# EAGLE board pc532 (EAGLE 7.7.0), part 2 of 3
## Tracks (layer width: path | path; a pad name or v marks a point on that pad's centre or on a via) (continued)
!SD0 (continued)
  Bottom 0.305: RES18.1 300.99,114.3 300.99,125.09 302.26,126.36 CONN16.2 300.99,130.81 300.99,133.35 288.93,145.41 286.38,145.41 CONN15.A14 284.48,149.86 283.21,151.13 283.21,163.83 284.48,165.1 CONN14.A14 284.48,170.18 283.21,171.45 283.21,184.15 284.48,185.42 CONN13.A14 284.48,190.5 283.21,191.77 283.21,204.47 284.48,205.74 CONN12.A14
!SD1
  Top 0.305: RES18.2 289.56,105.41 289.56,95.25 288.29,93.98 U57.9
  Bottom 0.305: RES18.2 299.72,115.57 CONN16.4 298.45,130.81 298.45,133.35 287.65,144.15 285.12,144.15 CONN15.A15 281.94,149.86 280.67,151.13 280.67,163.83 281.94,165.1 CONN14.A15 281.94,170.18 280.67,171.45 280.67,184.15 281.94,185.42 CONN13.A15 281.94,190.5 280.67,191.77 280.67,204.47 281.94,205.74 CONN12.A15
!SD2
  Route2 0.305: RES18.3 292.1,107.95 292.1,90.17 U57.8
  Bottom 0.305: RES18.3 297.18,115.57 CONN16.6 295.91,130.81 295.91,133.35 286.38,142.88 283.85,142.88 CONN15.A16 279.4,149.86 278.13,151.13 278.13,163.83 279.4,165.1 CONN14.A16 279.4,170.18 278.13,171.45 278.13,184.15 279.4,185.42 CONN13.A16 279.4,190.5 278.13,191.77 278.13,204.47 279.4,205.74 CONN12.A16
!SD3
  Route2 0.305: RES18.4 289.56,107.95 289.56,92.71 U57.7
  Bottom 0.305: RES18.4 294.64,115.57 CONN16.8 293.37,130.81 293.37,133.35 285.12,141.6 282.57,141.6 CONN15.A17 276.86,149.86 275.59,151.13 275.59,163.83 276.86,165.1 CONN14.A17 276.86,170.18 275.59,171.45 275.59,184.15 276.86,185.42 CONN13.A17 276.86,190.5 275.59,191.77 275.59,204.47 276.86,205.74 CONN12.A17
!SD4
  Route2 0.305: U57.6 294.64,90.17 294.64,110.49 293.37,111.76 288.29,111.76 RES18.5
  Bottom 0.305: RES18.5 292.1,115.57 CONN16.10 290.83,130.81 290.83,133.35 283.85,140.34 281.31,140.34 CONN15.A18 274.32,149.86 273.05,151.13 273.05,163.83 274.32,165.1 CONN14.A18 274.32,170.18 273.05,171.45 273.05,184.15 274.32,185.42 CONN13.A18 274.32,190.5 273.05,191.77 273.05,204.47 274.32,205.74 CONN12.A18
!SD5
  Top 0.305: RES18.6 287.02,105.41 287.02,88.27 288.93,86.36 U57.5
  Bottom 0.305: RES18.6 289.56,115.57 CONN16.12 288.29,130.81 288.29,133.35 282.57,139.06 280.04,139.06 CONN15.A19 271.78,149.86 270.51,151.13 270.51,163.83 271.78,165.1 CONN14.A19 271.78,170.18 270.51,171.45 270.51,184.15 271.78,185.42 CONN13.A19 271.78,190.5 270.51,191.77 270.51,204.47 271.78,205.74 CONN12.A19
!SD6
  Bottom 0.305: U57.4 294.64,87.63 294.64,100.33 RES18.13 287.02,107.95 282.57,107.95 281.94,108.58 281.94,109.86 287.02,114.94 CONN16.14 285.75,130.81 285.75,133.35 281.31,137.79 278.76,137.79 CONN15.A20 269.24,149.86 267.97,151.13 267.97,163.83 269.24,165.1 CONN14.A20 269.24,170.18 267.97,171.45 267.97,184.15 269.24,185.42 CONN13.A20 269.24,190.5 267.97,191.77 267.97,204.47 269.24,205.74 CONN12.A20
!SD7
  Bottom 0.305: U57.3 292.1,85.09 292.1,100.33 RES18.12 285.75,106.68 280.67,106.68 278.76,108.58 278.76,110.49 284.48,116.2 CONN16.16 283.21,130.81 283.21,133.35 280.04,136.53 277.5,136.53 CONN15.A21 266.7,149.86 265.43,151.13 265.43,163.83 266.7,165.1 CONN14.A21 266.7,170.18 265.43,171.45 265.43,184.15 266.7,185.42 CONN13.A21 266.7,190.5 265.43,191.77 265.43,204.47 266.7,205.74 CONN12.A21
!SD10
  Route2 0.305: CONN1.4 160.02,8.89 160.02,26.67 U41.39
  Bottom 0.305: U41.39 151.13,27.94 RES14.4
!SD20
  Top 0.305: U41.40 160.02,26.67 157.48,26.67 RES14.1
  Route2 0.305: CONN1.6 154.94,8.89 154.94,21.59 RES14.1
!SD30
  Route2 0.305: CONN1.8 152.4,8.89 152.4,21.59 RES14.2
  Bottom 0.305: U41.41 153.67,25.4 RES14.2
!SD40
  Route2 0.305: CONN1.10 149.86,8.89 149.86,21.59 RES14.3
  Bottom 0.305: U41.42 160.02,26.67 152.4,26.67 RES14.3
!SD50
  Bottom 0.305: CONN1.12 149.86,8.89 149.86,13.34 151.13,14.61 RES14.13 154.31,18.41 156.84,18.41 158.75,20.32 U41.44
!SD60
  Bottom 0.305: CONN1.14 147.32,8.89 147.32,13.34 148.59,14.61 RES14.12 153.03,19.68 155.57,19.68 157.48,21.59 160.02,21.59 U41.45
!SD70
  Top 0.305: U41.46 162.56,19.05 149.86,19.05 RES14.11
  Bottom 0.305: CONN1.16 144.78,8.89 144.78,13.34 146.05,14.61 RES14.11
!SDONE
  Top 0.305: U35.C6 157.48,163.83 157.48,170.81 156.84,171.45 R4.1 140.97,176.53 U24.J11
!SDP
  Bottom 0.305: CONN12.A22 264.16,205.74 262.89,204.47 262.89,191.77 264.16,190.5 CONN13.A22 264.16,185.42 262.89,184.15 262.89,171.45 264.16,170.18 CONN14.A22 264.16,165.1 262.89,163.83 262.89,151.13 264.16,149.86 CONN15.A22 276.23,135.25 278.76,135.25 280.67,133.35 280.67,130.81 CONN16.18 281.94,115.57 277.5,111.12 277.5,107.95 280.04,105.41 284.48,105.41 RES18.11 288.29,96.52 285.75,93.98 U57.11
!SDP0
  Bottom 0.305: CONN1.18 142.24,8.89 142.24,13.34 143.51,14.61 RES14.10 149.22,20.95 154.94,20.95 158.12,24.13 162.56,24.13 U41.47
!SIO
  Top 0.305: RES17.6 256.54,104.14 261.62,104.14 262.89,102.87 262.89,99.06 271.78,90.17 276.86,90.17 U57.19
  Bottom 0.305: RES17.6 241.3,119.38 CONN16.50 240.03,130.81 240.03,142.24 241.3,143.51 CONN15.A31 241.3,149.86 240.03,151.13 240.03,163.83 241.3,165.1 CONN14.A31 241.3,170.18 240.03,171.45 240.03,184.15 241.3,185.42 CONN13.A31 241.3,190.5 240.03,191.77 240.03,204.47 241.3,205.74 CONN12.A31
!SIO0
  Top 0.305: U41.33 123.19,35.56 RES12.6
  Bottom 0.305: CONN1.50 101.6,8.89 101.6,13.97 RES12.6
!SLOW
  Route15 0.305: U38.6 165.1,114.3 167.64,114.3 U37.19
!SLOWC
  Route15 0.305: U50.2 249.56,99.69 300.36,99.69 304.17,103.5 306.7,103.5 U58.4
!SLOWS  (via drill 0.33)
  Top 0.305: v188.59,104.78 184.78,108.58 166.37,108.58 165.1,109.86 165.1,111.76 160.66,116.2 158.12,116.2 U37.13
  Route15 0.305: U58.5 307.98,107.31 304.17,107.31 301.62,104.78 v188.59,104.78
!SMSG
  Bottom 0.305: U57.21 276.86,87.63 274.95,87.63 273.05,89.53 273.05,97.79 RES17.2 251.46,119.38 CONN16.42 250.19,130.81 250.19,142.24 251.46,143.51 CONN15.A27 251.46,149.86 250.19,151.13 250.19,163.83 251.46,165.1 CONN14.A27 251.46,170.18 250.19,171.45 250.19,184.15 251.46,185.42 CONN13.A27 251.46,190.5 250.19,191.77 250.19,204.47 251.46,205.74 CONN12.A27
!SMSG0
  Bottom 0.305: CONN1.42 111.76,8.89 111.76,12.06 114.3,14.61 114.3,16.51 RES12.2 129.54,31.75 154.94,31.75 157.48,34.29 160.02,34.29 U41.34
!SPC
  Bottom 0.305: U35.R9 185.42,171.45 177.8,171.45 175.26,173.99 148.59,173.99 147.32,175.26 135.89,175.26 U24.J10
!SREQ
  Bottom 0.305: U57.22 260.35,99.06 260.35,102.87 RES17.5 243.84,119.38 CONN16.48 242.57,130.81 242.57,142.24 243.84,143.51 CONN15.A30 243.84,149.86 242.57,151.13 242.57,163.83 243.84,165.1 CONN14.A30 243.84,170.18 242.57,171.45 242.57,184.15 243.84,185.42 CONN13.A30 243.84,190.5 242.57,191.77 242.57,204.47 243.84,205.74 CONN12.A30
!SREQ0
  Route15 0.305: RES12.5 113.03,35.56 120.65,43.18 U41.27
  Bottom 0.305: CONN1.48 104.14,8.89 104.14,13.97 RES12.5
!SRST
  Bottom 0.305: U57.18 275.59,97.79 RES17.1 254,119.38 CONN16.40 252.73,130.81 252.73,142.24 254,143.51 CONN15.A26 254,149.86 252.73,151.13 252.73,163.83 254,165.1 CONN14.A26 254,170.18 252.73,171.45 252.73,184.15 254,185.42 CONN13.A26 254,190.5 252.73,191.77 252.73,204.47 254,205.74 CONN12.A26
!SRST0
  Top 0.305: RES12.11 120.65,20.32 123.83,20.32 137.79,34.29 160.02,34.29 U41.36
  Bottom 0.305: CONN1.40 114.3,8.89 114.3,12.06 115.57,13.34 RES12.11
!SSEL
  Top 0.305: U57.14 281.94,90.17 281.94,92.08 280.04,93.98 274.32,93.98 RES17.3
  Bottom 0.305: RES17.3 248.92,119.38 CONN16.44 247.65,130.81 247.65,142.24 248.92,143.51 CONN15.A28 248.92,149.86 247.65,151.13 247.65,163.83 248.92,165.1 CONN14.A28 248.92,170.18 247.65,171.45 247.65,184.15 248.92,185.42 CONN13.A28 248.92,190.5 247.65,191.77 247.65,204.47 248.92,205.74 CONN12.A28
!SSEL0
  Route15 0.305: RES12.3 118.11,38.1 120.65,40.64 U41.29
  Bottom 0.305: CONN1.44 109.22,8.89 109.22,12.06 111.76,14.61 111.76,16.51 RES12.3
!TXD0
  Top 0.305: U47.14 U48.33
!TXD1
  Route2 0.305: U48.13 201.93,26.67 201.93,16.51 U49.14
!TXD2
  Top 0.305: U51.14 U52.33
!TXD3
  Route2 0.305: U52.13 236.22,26.67 236.22,16.51 U53.14
!TXD4
  Top 0.305: U54.14 U55.33
!TXD5
  Route2 0.305: U55.13 270.51,26.67 270.51,16.51 U56.14
!TXD6
  Top 0.305: U59.14 U60.33
!TXD7
  Route2 0.305: U60.13 304.8,26.67 304.8,16.51 U61.14
!WEA
  Route2 0.305: U18.6 58.42,73.66 RES7.5
!WEAB
  Route2 0.305: U18.9 63.5,66.04 U18.5
  Bottom 0.305: U18.5 65.41,69.22 107.95,69.22 117.47,78.74 117.47,88.27 120.02,90.81 126.36,90.81 U30.11
!WEAR
  Route2 0.305: U6.21 50.8,139.7 50.8,127 U8.21 50.8,124.46 50.8,111.76 U10.21 50.8,109.22 50.8,96.52 U12.21 50.8,93.98 50.8,85.09 RES7.6
!WEB
  Route2 0.305: RES7.7 53.34,68.58 U18.8
!WEBR
  Route2 0.305: RES7.8 49.53,81.28 U13.21 49.53,92.71 48.26,93.98 48.26,96.52 49.53,97.79 U11.21 49.53,107.95 48.26,109.22 48.26,111.76 49.53,113.03 U9.21 49.53,123.19 48.26,124.46 48.26,127 49.53,128.27 U7.21
!WR
  Top 0.305: U46.31 231.14,63.5 252.09,63.5 255.27,60.33 255.27,31.75 252.73,29.21 233.68,29.21 U52.9 | U38.18 172.72,99.06 172.72,57.15 170.18,54.61 170.18,44.45 U41.21
  Route2 0.305: U41.21 168.91,39.37 179.07,29.21 196.85,29.21 U48.9
  Route15 0.305: U48.9 199.39,26.67 231.14,26.67 U52.9 233.68,26.67 265.43,26.67 U55.9 267.97,26.67 299.72,26.67 U60.9 | U46.31 232.41,74.93 279.4,74.93 U57.32
+5V
  pour Power (rank 6): 0,215.9 0,58.42 12.7,58.42 12.7,0 342.9,0 342.9,215.9
+12V
  Top 0.813: CONN12.B9 297.18,210.82 323.21,210.82 327.02,207.01 327.02,198.12 | 327.02,198.12 300.99,198.12 297.18,194.31 CONN13.B9 | 327.02,198.12 327.02,180.34 | 327.02,180.34 C68.+ | 327.02,180.34 327.02,177.8 | 327.02,177.8 300.99,177.8 297.18,173.99 CONN14.B9 | 327.02,177.8 327.02,157.48 | 327.02,157.48 300.99,157.48 297.18,153.67 CONN15.B9 | 327.02,157.48 327.02,92.08 322.58,87.63 322.58,71.75 325.75,68.58 325.75,45.72 323.85,43.81 323.85,31.11 325.12,29.84 325.12,14.61 322.58,12.06 313.06,12.06 310.31,9.32 CONN11.P8-3
  Route15 0.305: 275.59,59.69 U54.1
  Route15 0.406: U56.1 278.13,24.13 309.88,24.13 U61.1 311.15,20.32 309.88,19.05 309.88,12.7 310.31,12.27 CONN11.P8-3 | U49.1 209.55,24.13 241.3,24.13 U53.1 248.92,16.51 248.92,13.97 252.73,10.16 C59.+ | U47.1 209.55,59.69 241.3,59.69 U51.1 243.84,59.69 275.59,59.69 | U54.1 278.13,59.69 309.88,59.69 U59.1
  Route15 0.813: C59.+ 260.99,10.16 262.89,8.26 265.43,8.26 270.51,3.17 308.61,3.17 310.31,4.88 CONN11.P8-3
  Bottom 0.406: U61.1 316.23,27.94 316.23,53.34 U59.1
+V  (via drill 0.33)
  Top 0.305: U35.D11 U35.C11 | U35.C11 U35.B11 | U35.B11 U35.A11 | U35.C12 U35.C11 | U35.C11 U35.C10 | U35.B12 U35.B11 | U35.B11 U35.B10 | U32.4 125.73,68.58 U32.10 | U31.4 129.54,82.55 134.62,82.55 U31.1 | v226.06,111.76 226.06,103.5 228.6,100.97 v228.6,92.71
  Route2 0.305: U35.N12 177.16,177.8 174.62,175.26 U35.D11 | U35.S14 205.74,182.88 224.79,163.83 224.79,144.78 | 224.79,144.78 224.79,142.24 U43.22 | 224.79,144.78 227.33,142.24 227.33,113.03 v226.06,111.76 | U30.10 127,87.63 127,85.09 U31.4 127,82.55 127,72.39 U32.4 | U46.28 220.34,70.48 220.34,74.93 224.79,79.38 224.79,84.45 228.6,88.27 v228.6,92.71 | RES13.2 179.07,86.36 v179.07,106.68 179.07,132.08 175.26,135.89 173.99,135.89 U36.2
  Route15 0.305: U30.5 127,95.25 127,90.17 U30.10 | U35.R14 185.42,181.61 183.51,181.61 182.88,180.97 182.88,179.07 | 182.88,179.07 U35.N12 | U35.B12 U35.B13 | U35.D11 160.02,173.99 160.02,163.83 U35.D6 | RES13.2 162.56,72.39 160.02,72.39 RES13.4 RES13.5 154.94,72.39 129.54,72.39 U32.4 | v179.07,106.68 203.84,106.68 205.74,108.58 222.88,108.58 v226.06,111.76 | U50.1 245.11,92.71 v228.6,92.71 | U24.B7 125.73,195.58 125.73,201.93 128.27,204.47 137.16,204.47 149.86,191.77 149.86,184.15 U35.A14 | 182.88,179.07 U35.P12
  Bottom 0.305: U26.1 135.89,151.13 135.89,156.21 140.97,161.29 157.48,161.29 U35.D6 | U33.6 U32.10 | U35.R14 U35.S14 | U35.B13 U35.A13 U35.A14 | U24.A5 123.19,195.58 | 123.19,195.58 125.73,195.58 U24.B7 | U24.B5 123.19,195.58
-12V
  Top 0.406: U61.8 292.1,24.13 292.1,57.15 U59.8
  Route2 0.61: 304.17,3.17 306.35,5.36 CONN11.P8-4
  Route2 0.635: C60.- 268.61,5.08 270.51,3.17 304.17,3.17
  Route15 0.406: U56.8 260.35,21.59 290.83,21.59 | 290.83,21.59 292.1,21.59 U61.8 | U47.8 191.77,57.15 223.52,57.15 U51.8 226.06,57.15 257.81,57.15 U54.8 260.35,57.15 292.1,57.15 U59.8 | 290.83,21.59 290.83,15.24 293.37,12.7 302.26,12.7 306.35,8.61 CONN11.P8-4
  Bottom 0.406: U56.8 257.81,21.59 226.06,21.59 U53.8 223.52,21.59 191.77,21.59 U49.8
  Bottom 0.813: CONN12.B7 302.26,210.82 323.21,210.82 327.02,207.01 327.02,198.12 | 327.02,198.12 305.44,198.12 302.26,194.94 CONN13.B7 | 327.02,198.12 327.02,194.31 | 327.02,194.31 C67.- | 327.02,194.31 327.02,177.8 | 327.02,177.8 306.07,177.8 302.26,173.99 CONN14.B7 | 327.02,177.8 327.02,157.48 | 327.02,157.48 306.07,157.48 302.26,153.67 CONN15.B7 | 327.02,157.48 327.02,92.08 322.58,87.63 322.58,71.12 331.47,62.23 331.47,15.88 327.66,12.06 309.25,12.06 306.35,9.17 CONN11.P8-4
_STERM
  Top 0.813: D3.A F2.1
_STERM0
  Top 0.813: D1.A F1.1
A0  (via drill 0.33)
  Route2 0.305: U44.10 204.47,132.08 204.47,98.42 v203.84,97.79
  Route15 0.305: U35.R6 187.96,161.29 190.5,161.29 201.93,149.86 201.93,139.7 205.74,135.89 U44.10
  Bottom 0.305: v203.84,97.79 214.63,97.79 U45.3
A1
  Route2 0.305: U45.5 210.82,97.79 207.01,101.6 207.01,132.08 U44.9
  Route15 0.305: U35.S5 191.77,157.48 191.77,147.32 204.47,134.62 204.47,132.72 205.1,132.08 207.01,132.08 U44.9
A2
  Route2 0.305: U27.2 142.88,141.6 142.88,151.76 149.86,158.75 165.1,158.75 167.64,161.29 182.88,161.29 U35.P6 | U44.8 210.82,129.54 212.09,128.27 212.09,92.71 U45.9
  Route15 0.305: U44.8 204.47,139.7 204.47,149.86 190.5,163.83 185.42,163.83 U35.P6
A3
  Top 0.305: U27.5 133.35,139.7 138.43,139.7 146.69,147.96 164.47,147.96 165.1,148.59 165.1,156.21 167.64,158.75 187.96,158.75 U35.S4
  Route2 0.305: U45.11 217.17,92.71 217.17,101.6 214.63,104.14 214.63,129.54 213.36,130.81 U44.7
  Route15 0.305: U35.S4 190.5,156.21 190.5,147.32 201.93,135.89 201.93,132.08 203.2,130.81 210.82,130.81 U44.7
A4  (via drill 0.33)
  Top 0.305: U27.11 125.73,129.54 128.27,132.08 138.43,132.08 140.34,133.99 140.34,135.25 141.6,136.53 143.51,136.53 144.15,137.16 144.15,143.51 147.32,146.69 v159.38,146.69
  Route2 0.305: U45.13 219.71,90.17 219.71,129.54 U44.6
  Route15 0.305: v159.38,146.69 163.19,146.69 165.1,148.59 165.1,156.21 167.64,158.75 185.42,158.75 U35.R5 187.96,158.75 187.96,148.59 199.39,137.16 199.39,132.08 201.93,129.54 212.09,129.54 U44.6
A5  (via drill 0.33)
  Top 0.305: v187.96,142.24 187.96,137.16 181.61,130.81 181.61,127 177.8,123.19 163.83,123.19 162.56,121.92 146.05,121.92 144.15,123.83 136.53,123.83 U27.14
  Route2 0.305: U44.5 222.25,129.54 222.25,114.3 220.98,113.03 U45.1
  Bottom 0.305: U35.S3 187.96,153.67 v187.96,142.24 190.5,139.7 212.09,139.7 U44.5
A6  (via drill 0.33)
  Top 0.305: v155.57,142.88 153.67,140.97 v145.41,140.97
  Route2 0.305: U33.3 132.08,57.15 130.18,57.15 129.54,57.78 129.54,59.69 132.08,62.23 132.08,64.77 134.62,67.31 134.62,73.03 132.08,75.56 132.08,85.09 129.54,87.63 129.54,97.79 132.08,100.33 132.08,104.14 134.62,106.68 134.62,115.57 135.89,116.84 U28.2
  Route15 0.305: U28.2 140.34,126.36 140.34,128.91 144.15,132.72 144.15,139.7 v145.41,140.97 | v155.57,142.88 155.57,146.05 157.48,147.96 161.93,147.96 162.56,148.59 162.56,156.21 167.64,161.29 182.88,161.29 U35.P5
  Bottom 0.305: U44.4 214.63,139.7 214.63,142.24 213.36,143.51 193.04,143.51 191.77,144.78 191.77,157.48 190.5,158.75 185.42,158.75 U35.P5
A7  (via drill 0.33)
  Top 0.305: v156.84,144.78 v147.32,144.78
  Route15 0.305: v156.84,144.78 163.83,144.78 167.64,148.59 167.64,155.57 168.28,156.21 185.42,156.21 U35.R4 | v147.32,144.78 146.05,144.78 140.34,139.06 140.34,133.99 138.43,132.08 133.35,132.08 129.54,128.27 129.54,123.19 U28.5
  Bottom 0.305: U35.R4 185.42,156.21 185.42,148.59 186.69,147.32 186.69,140.97 189.23,138.43 212.09,138.43 214.63,135.89 214.63,132.08 215.9,130.81 220.98,130.81 U44.3
A8  (via drill 0.33)
  Top 0.305: U44.25 222.25,116.84 224.16,116.84 224.79,117.47 224.79,119.38 222.25,121.92 222.25,142.24 219.71,144.78 196.85,144.78 U35.S2 | v182.25,138.43 v189.23,145.41
  Route15 0.305: v182.25,138.43 175.9,132.08 175.9,130.18 174.62,128.91 161.93,128.91 U37.7
  Bottom 0.305: U35.S2 190.5,151.13 190.5,146.69 v189.23,145.41 | U28.11 127,113.03 129.54,113.03 132.08,110.49 132.08,107.95 133.35,106.68 139.06,106.68 140.34,107.95 140.34,110.49 141.6,111.76 152.4,111.76 157.48,116.84 157.48,124.46 U37.7
A9  (via drill 0.33)
  Top 0.305: U28.14 135.89,116.84 144.78,116.84 148.59,120.65 179.07,120.65 v181.61,123.19 | U35.R3 187.96,153.67 190.5,153.67 198.12,146.05 220.98,146.05 224.79,142.24 224.79,121.92 227.33,119.38 227.33,117.47 225.43,115.57 220.98,115.57 U44.24
  Bottom 0.305: v181.61,123.19 186.69,123.19 195.58,114.3 214.63,114.3 U44.24
A10  (via drill 0.33)
  Top 0.305: v182.88,129.54 182.88,121.92 180.34,119.38 149.86,119.38 142.24,111.76 138.43,111.76 U29.2
  Bottom 0.305: U44.21 204.47,124.46 190.5,124.46 185.42,129.54 184.15,129.54 | 184.15,129.54 v182.88,129.54 | 184.15,129.54 184.15,147.32 182.88,148.59 182.88,156.21 U35.P4
A11  (via drill 0.33)
  Top 0.305: U29.5 130.18,107.31 142.88,107.31 144.15,106.05 148.59,106.05 149.86,107.31 v173.99,107.31
  Bottom 0.305: U44.23 213.36,115.57 208.28,115.57 207.01,116.84 207.01,119.38 204.47,121.92 190.5,121.92 186.69,125.73 180.34,125.73 | 180.34,125.73 180.34,110.49 177.16,107.31 v173.99,107.31 | U35.N4 180.34,156.21 180.34,125.73
A12  (via drill 0.33)
  Top 0.305: U35.R2 185.42,153.67 185.42,155.57 186.06,156.21 190.5,156.21 199.39,147.32 222.25,147.32 227.33,142.24 227.33,134.62 U44.2
  Route2 0.305: U29.11 132.08,107.95 132.08,115.57 134.62,118.11 134.62,123.19 135.89,124.46 143.51,124.46 146.69,127.64 | 146.69,127.64 J1.3 | 146.69,127.64 147.32,128.27 153.67,128.27 154.94,129.54 154.94,131.44 155.57,132.08 165.1,132.08 v166.37,133.35
  Route15 0.305: U35.R2 185.42,151.13 185.42,149.22 179.71,143.51 171.45,143.51 167.64,139.7 167.64,135.89 166.37,134.62 v166.37,133.35
A13
  Top 0.305: U36.3 168.91,140.97 175.26,147.32 186.69,147.32 U35.S1 195.58,143.51 218.44,143.51 219.71,142.24 219.71,121.92 U44.26
  Route2 0.305: U36.3 165.1,134.62 157.48,134.62 156.21,133.35 153.67,133.35 152.4,132.08 152.4,130.18 151.76,129.54 150.5,129.54 147.96,132.08 128.27,132.08 U27.6
A14  (via drill 0.33)
  Top 0.305: U36.4 169.54,135.25 v182.25,135.25 | U27.10 123.19,129.54 127,133.35 131.44,133.35 132.08,133.99 132.08,135.89 134.62,138.43 v142.88,138.43
  Route2 0.305: U35.N3 180.34,156.21 149.86,156.21 144.15,150.5 144.15,139.7 v142.88,138.43
  Route15 0.305: U35.N3 180.34,153.67 180.34,149.22 175.9,144.78 171.45,144.78 166.37,139.7 U36.4 | v182.25,135.25 187.96,135.25 200.03,123.19 220.98,123.19 U44.27
A15  (via drill 0.33)
  Top 0.305: U27.13 132.08,128.27 153.67,128.27 154.94,129.54 v154.94,134.62 | U36.5 173.99,148.59 185.42,148.59 U35.R1
  Route2 0.305: v154.94,134.62 156.21,135.89 161.29,135.89 U36.5
A16
  Route2 0.305: U35.P1 184.15,148.59 176.53,140.97 163.83,140.97 U36.6
  Bottom 0.305: U28.3 134.62,123.19 134.62,135.89 138.43,139.7 160.02,139.7 U36.6
A17
  Route15 0.305: U35.M3 177.8,153.67 177.8,151.76 177.16,151.13 175.9,151.13 175.26,150.5 175.26,149.22 173.35,147.32 171.45,147.32 165.1,140.97 161.29,140.97 U36.7
  Bottom 0.305: U28.6 128.27,119.38 138.43,119.38 140.34,121.28 140.34,129.54 145.41,134.62 152.4,134.62 153.67,135.89 156.21,135.89 U36.7
A18  (3 unrouted)
  Top 0.305: U36.8 154.94,139.7 150.5,139.7 149.86,139.06 149.86,135.89 148.59,134.62 144.78,134.62 140.97,130.81 129.54,130.81 127,128.27 127,118.11 U28.10
  Route2 0.305: U36.8 163.19,145.41 176.53,145.41 180.97,149.86 U35.N2
A19
  Top 0.305: U28.13 130.81,116.84 129.54,118.11 129.54,128.27 130.81,129.54 147.32,129.54 153.67,135.89 U36.9
  Route2 0.305: U36.9 154.94,137.16 160.02,137.16 160.02,139.7 164.47,144.15 177.8,144.15 182.88,149.22 182.88,151.13 U35.N1
A20
  Route2 0.305: U35.M1 175.9,146.69 163.19,146.69 157.48,140.97 153.67,140.97 152.4,139.7 152.4,134.62 151.13,133.35 U36.11
  Bottom 0.305: U29.3 137.16,113.03 137.16,115.57 140.34,118.75 141.6,118.75 144.78,121.92 144.78,124.46 U36.11
A21
  Route15 0.305: U29.6 128.27,111.76 152.4,111.76 157.48,116.84 157.48,127 U36.12 157.48,134.62 157.48,139.7 160.02,142.24 165.1,142.24 171.45,148.59 172.09,148.59 172.72,149.22 172.72,153.03 173.35,153.67 175.26,153.67 U35.L2
A22
  Route2 0.305: U38.9 153.67,114.3 154.94,115.57 154.94,127 156.21,128.27 U36.13
  Route15 0.305: U36.13 160.02,134.62 161.93,134.62 165.1,137.79 165.1,139.7 171.45,146.05 173.99,146.05 176.53,148.59 U35.L1
  Bottom 0.305: U38.9 151.13,107.95 J2.3 142.24,103.5 125.09,103.5 U29.10
A23
  Route2 0.305: J1.1 146.69,137.79 156.84,147.96 171.45,147.96 172.72,149.22 172.72,151.13 U35.K2
A24  (via drill 0.33)
  Top 0.305: v158.12,143.51 157.48,142.88 157.48,132.08 U36.14
  Route15 0.305: v158.12,143.51 164.47,143.51 170.18,149.22 170.18,153.67 U35.J3
  Bottom 0.305: U36.14 157.48,129.54 152.4,129.54 146.69,123.83 J2.1
A27  (via drill 0.33)
  Top 0.305: U37.5 163.83,128.27 162.56,129.54 162.56,140.97 168.91,147.32 U35.H1
  Route2 0.305: U40.9 156.21,60.96 153.67,60.96 152.4,62.23 v152.4,100.33
  Bottom 0.305: v152.4,100.33 152.4,103.5 155.57,106.68 157.48,106.68 160.02,109.22 160.02,120.65 163.83,124.46 U37.5
A28
  Bottom 0.305: U35.H2 167.64,151.13 165.74,151.13 165.1,150.5 165.1,127 U37.4
A29
  Bottom 0.305: U37.3 168.91,128.27 167.64,129.54 167.64,148.59 U35.G1
A30
  Bottom 0.305: U35.F1 162.56,151.13 162.56,153.03 163.19,153.67 169.54,153.67 170.18,153.03 170.18,130.18 171.45,128.91 U37.2
A31
  Top 0.305: U35.G2 167.64,151.13 167.64,148.59 160.02,140.97 160.02,129.54 162.56,127 162.56,125.09 163.19,124.46 172.72,124.46 U37.1
ASEL
  Route2 0.305: U29.1 137.16,110.49 137.16,120.65 U28.1
  Route15 0.305: U31.5 129.54,87.63 129.54,90.81 132.08,93.34 132.08,102.87 U29.1
  Bottom 0.305: U28.1 137.16,123.19 137.16,133.35 U27.1
BA0  (via drill 0.33)
  Top 0.305: U60.2 297.18,36.83 297.18,54.61 294.64,57.15 294.64,79.38 294,80.01 287.02,80.01 284.48,77.47 284.48,74.93 U57.33 | U46.22 200.66,66.04 198.12,66.04 191.77,59.69 191.77,46.99 194.31,44.45 194.31,36.83 U48.2
  Route2 0.305: v203.84,95.25 201.93,93.34 201.93,69.85 U46.22
  Route15 0.305: U60.2 294.64,36.83 262.89,36.83 U55.2 260.35,36.83 228.6,36.83 U52.2 226.06,36.83 194.31,36.83 U48.2 190.5,33.02 190.5,28.57 186.06,24.13 180.34,24.13 U41.59
  Bottom 0.305: U45.4 212.09,95.25 v203.84,95.25
BA1  (via drill 0.33)
  Top 0.305: v210.82,45.72 v215.9,40.64
  Route2 0.305: v215.9,40.64 v215.9,35.56 | v210.82,45.72 210.82,63.5 U46.23 205.74,81.92 204.47,83.19 204.47,90.17 208.28,93.98 U45.6
  Route15 0.305: U57.36 287.02,74.93 298.45,74.93 313.69,59.69 313.69,48.26 316.23,45.72 316.23,33.02 314.96,31.75 297.18,31.75 U60.4
  Bottom 0.305: U60.4 294.64,34.29 262.89,34.29 U55.4 260.35,34.29 228.6,34.29 U52.4 226.06,34.29 215.9,34.29 | 215.9,34.29 194.31,34.29 U48.4 | v215.9,35.56 215.9,34.29
BA2  (via drill 0.33)
  Top 0.305: v213.36,48.26 213.36,45.09 214,44.45 215.9,44.45 218.44,41.91 v218.44,33.02 | U57.37 287.02,72.39 282.57,72.39 281.94,73.03 281.94,78.74 285.75,82.55 302.26,82.55 323.85,60.96 323.85,46.35 321.94,44.45 321.94,31.11 320.04,29.21 297.18,29.21 U60.6
  Route2 0.305: v213.36,48.26 213.36,63.5 U46.24 208.28,81.92 207.01,83.19 207.01,87.63 U45.8
  Route15 0.305: v218.44,33.02 218.44,31.75 | 218.44,31.75 226.06,31.75 U52.6 228.6,31.75 260.35,31.75 U55.6 262.89,31.75 294.64,31.75 U60.6 | 218.44,31.75 194.31,31.75 U48.6
BA3  (via drill 0.33)
  Top 0.305: v214.63,45.72 217.17,45.72 219.71,43.18 219.71,35.56 v222.25,33.02
  Route2 0.305: U45.10 209.55,87.63 209.55,83.19 210.82,81.92 U46.25 210.82,67.31 214.63,63.5 v214.63,45.72 | v222.25,33.02 227.33,27.94 U52.7
  Bottom 0.305: U60.7 297.18,26.67 265.43,26.67 U55.7 262.89,26.67 231.14,26.67 U52.7 228.6,26.67 196.85,26.67 U48.7
BA4
  Route2 0.305: U46.26 217.17,72.39 217.17,87.63 U45.12
  Bottom 0.305: U46.26 212.09,67.31 176.53,67.31 170.18,60.96 170.18,57.78 169.54,57.15 139.7,57.15 U33.1
BA5
  Bottom 0.305: U33.2 135.89,59.05 137.79,60.96 140.34,60.96 149.86,70.48 149.86,73.03 157.48,80.64 164.47,80.64 169.54,85.72 179.07,85.72 183.51,90.17 213.36,90.17 218.44,95.25 U45.2
BANKS  (via drill 0.33)
  Top 0.305: U19.8 69.85,57.15 73.03,57.15 77.47,52.7 v77.47,52.07
  Route15 0.305: v77.47,52.07 77.47,48.26 78.74,46.99 U20.4
  Bottom 0.305: J2.2 140.97,104.78 123.83,104.78 121.92,102.87 121.92,100.33 121.28,99.69 118.75,99.69 101.6,82.55 99.69,82.55 97.79,80.64 97.79,78.74 92.71,73.66 64.14,73.66 62.23,71.75 62.23,69.85 67.31,64.77 67.31,59.69 U19.8
BCLK  (via drill 0.33)
  Route2 0.305: U39.1 172.72,97.79 172.72,109.22 U38.1
  Route15 0.305: U39.1 176.53,93.98 180.97,93.98 183.51,91.44 228.6,91.44 U50.9 | 27.94,35.56 26.04,35.56 R3.2 | 27.94,35.56 83.19,35.56 85.09,37.47 85.09,41.27 86.36,42.55 U20.1 88.9,48.26 101.6,48.26 121.28,67.94 127.64,67.94 U32.3 | v161.29,162.56 161.29,175.26 160.02,176.53 157.48,176.53 | 157.48,176.53 149.86,176.53 148.59,177.8 148.59,191.13 136.53,203.2 131.44,203.2 129.54,201.29 U24.A8 | 157.48,176.53 157.48,168.91 U35.D8 157.48,166.37 149.86,166.37 147.96,164.47 C24.1 | U16.11 27.94,35.56
  Bottom 0.305: U39.1 173.99,92.08 172.72,90.81 165.74,90.81 165.1,90.17 165.1,87 161.29,83.19 156.21,83.19 142.88,69.85 132.08,69.85 U32.3 | U38.1 175.9,112.39 175.9,145.41 175.26,146.05 175.26,156.21 170.18,161.29 162.56,161.29 v161.29,162.56
BD0
  Top 0.305: U43.20 217.17,142.24 200.03,142.24 199.39,141.6 199.39,137.16 200.66,135.89 | 200.66,135.89 U44.11 | 200.66,135.89 194.31,135.89 191.77,133.35 191.77,95.25 U46.19
  Route2 0.305: U46.19 203.2,71.12 204.47,69.85 204.47,67.31 209.55,62.23 209.55,44.45 U48.28 | U57.2 292.1,82.55 289.56,82.55 284.48,77.47 284.48,72.39 279.4,67.31 U55.28
  Bottom 0.305: U60.28 312.42,44.45 280.67,44.45 U55.28 278.13,44.45 246.38,44.45 U52.28 243.84,44.45 212.09,44.45 U48.28 209.55,44.45 185.42,44.45 U41.9 182.88,44.45 172.72,44.45 U41.18 170.18,46.99 119.38,46.99 114.3,41.91 80.01,41.91 U20.20
BD1
  Top 0.305: U46.18 204.47,85.09 203.84,85.09 193.04,95.89 193.04,132.72 194.94,134.62 199.39,134.62 U44.12
  Route15 0.305: U60.18 316.23,30.48 317.5,31.75 317.5,58.42 294.64,81.28 U57.44
  Bottom 0.305: U46.18 218.44,71.12 256.54,71.12 260.35,67.31 292.1,67.31 297.81,73.03 297.81,78.11 294.64,81.28 U57.44 | U20.21 81.28,40.64 114.94,40.64 116.2,41.91 172.72,41.91 U41.17 178.44,38.73 | U60.18 312.42,29.21 280.67,29.21 U55.18 278.13,29.21 246.38,29.21 U52.18 243.84,29.21 212.09,29.21 U48.18 209.55,29.21 180.34,29.21 178.44,31.11 178.44,38.73 | U41.8 179.71,38.73 178.44,38.73 | U44.12 204.47,129.54 223.52,129.54 224.79,130.81 224.79,133.99 224.16,134.62 222.25,134.62 U43.19
BD2
  Top 0.305: U44.13 194.31,129.54 194.31,96.52 204.47,86.36 205.74,86.36 U46.17
  Route2 0.305: U55.27 278.13,41.91 280.67,41.91 281.94,43.18 281.94,67.31 287.02,72.39 287.02,77.47 288.29,78.74 U57.43
  Route15 0.305: U41.16 175.26,46.99 182.25,46.99 182.88,46.35 182.88,41.91 U41.7 | U44.13 198.12,132.08 201.93,128.27 213.36,128.27 217.17,132.08 217.17,135.89 213.36,139.7 U43.18
  Bottom 0.305: U20.19 78.74,43.18 105.41,43.18 110.49,48.26 171.45,48.26 U41.16 | U41.7 185.42,41.91 207.01,41.91 U48.27 209.55,41.91 241.3,41.91 U52.27 243.84,41.91 275.59,41.91 U55.27 278.13,41.91 309.88,41.91 U60.27 | U57.43 292.1,80.01 294,80.01 296.55,77.47 296.55,73.66 291.46,68.58 261.62,68.58 256.54,73.66 218.44,73.66 U46.17
BD3  (via drill 0.33)
  Top 0.305: U46.16 207.01,87.63 205.1,87.63 195.58,97.16 U44.15 | v151.76,39.37 172.72,39.37 U41.15 | U57.42 292.1,77.47 292.1,69.85 290.83,68.58 290.83,41.91 280.67,31.75 278.13,31.75 U55.19
  Route2 0.305: U44.15 194.31,119.38 194.31,139.06 200.03,144.78 207.01,144.78 U43.17 | U41.15 U41.6
  Bottom 0.305: U46.16 219.71,74.93 257.81,74.93 262.89,69.85 290.83,69.85 295.27,74.3 295.27,76.83 U57.42 | U41.6 179.71,36.2 179.71,33.02 180.97,31.75 207.01,31.75 U48.19 209.55,31.75 241.3,31.75 U52.19 243.84,31.75 275.59,31.75 U55.19 278.13,31.75 309.88,31.75 U60.19 | v151.76,39.37 150.5,40.64 116.84,40.64 115.57,39.37 82.55,39.37 U20.22
BD4
  Top 0.305: U44.16 198.12,96.52 203.2,91.44 210.19,91.44 212.09,89.53 212.09,85.09 U46.15 | U41.5 182.88,39.37 182.88,43.81 182.25,44.45 177.8,44.45 U41.14
  Route2 0.305: U44.16 196.85,119.38 196.85,140.34 200.03,143.51 205.74,143.51 U43.16 | U55.26 281.94,40.64 284.48,43.18 284.48,66.04 289.56,71.12 289.56,74.93 U57.41 | U48.26 209.55,39.37 185.42,39.37 U41.5
  Bottom 0.305: U46.15 220.98,76.2 259.08,76.2 264.16,71.12 290.19,71.12 292.1,73.03 292.1,74.93 U57.41 | U60.26 312.42,39.37 280.67,39.37 U55.26 278.13,39.37 246.38,39.37 U52.26 243.84,39.37 212.09,39.37 U48.26 | U41.14 172.72,49.53 109.86,49.53 104.78,44.45 77.47,44.45 U20.18
BD5
  Top 0.305: U44.17 201.93,116.84 201.93,94.61 203.84,92.71 211.46,92.71 214.63,89.53 214.63,85.09 U46.14 | U41.13 179.07,38.1 U41.4
  Route2 0.305: U57.40 293.37,69.85 290.83,67.31 290.83,34.29 | U41.4 182.88,36.83 204.47,36.83 207.01,34.29 209.55,34.29 U48.20 212.09,34.29 243.84,34.29 U52.20 246.38,34.29 278.13,34.29 U55.20 280.67,34.29 290.83,34.29 | 290.83,34.29 312.42,34.29 U60.20 | U44.17 199.39,119.38 199.39,141.6 200.03,142.24 204.47,142.24 U43.15
  Bottom 0.305: U57.40 292.1,77.47 271.78,77.47 270.51,78.74 220.98,78.74 U46.14
BD6  (via drill 0.33)
  Top 0.305: U46.13 219.71,82.55 219.71,63.5 220.98,62.23 v220.98,40.64 | U41.3 185.42,36.83 185.42,43.81 182.25,46.99 180.34,46.99 U41.12
  Route2 0.305: U57.39 290.83,69.85 289.56,68.58 289.56,45.72 283.21,39.37 278.13,39.37 U55.25 | U46.13 222.25,87.63 v222.25,110.49 | U44.18 201.93,119.38 201.93,139.7 U43.14
  Route15 0.305: U48.25 209.55,39.37 220.98,39.37 | 220.98,39.37 v220.98,40.64 | 220.98,39.37 241.3,39.37 U52.25 243.84,39.37 275.59,39.37 U55.25 278.13,39.37 309.88,39.37 U60.25 | v222.25,110.49 220.98,110.49 214.63,116.84 214.63,119.38 213.36,120.65 205.74,120.65 U44.18
  Bottom 0.305: U41.3 187.96,35.56 191.77,39.37 207.01,39.37 U48.25
BD7  (via drill 0.33)
  Top 0.305: U43.13 200.66,139.7 204.47,135.89 204.47,119.38 U44.19 207.01,116.84 207.01,95.89 208.91,93.98 215.26,93.98 219.71,89.53 219.71,85.09 U46.12 220.98,80.01 222.25,78.74 v222.25,35.56 | U55.21 278.13,34.29 280.67,34.29 289.56,43.18 289.56,74.93 U57.38
  Route2 0.305: U41.2 182.88,34.29 204.47,34.29 205.74,33.02 U48.21
  Route15 0.305: U60.21 309.88,34.29 278.13,34.29 U55.21 275.59,34.29 243.84,34.29 U52.21 241.3,34.29 222.25,34.29 | 222.25,34.29 209.55,34.29 U48.21 | U41.11 179.71,41.27 179.71,34.92 U41.2 | v222.25,35.56 222.25,34.29
CLK
  Top 0.305: U25.8 123.19,158.75 159.38,158.75 160.02,159.38 160.02,171.45 U35.D10
CTS0
  Top 0.305: U47.4 204.47,54.61 213.36,54.61 215.9,52.07 218.44,52.07 CONN3.6
CTS1
  Top 0.305: U49.4 204.47,19.05 218.44,19.05 CONN4.6
CTS2
  Top 0.305: U51.4 238.76,54.61 247.65,54.61 250.19,52.07 252.73,52.07 CONN5.6
CTS3
  Top 0.305: U53.4 238.76,19.05 252.73,19.05 CONN6.6
CTS4
  Top 0.305: U54.4 273.05,54.61 281.94,54.61 284.48,52.07 287.02,52.07 CONN7.6
CTS5
  Top 0.305: U56.4 273.05,19.05 287.02,19.05 CONN8.6
CTS6
  Top 0.305: U59.4 307.34,54.61 316.23,54.61 318.77,52.07 321.31,52.07 CONN9.6
CTS7
  Top 0.305: U61.4 307.34,19.05 321.31,19.05 CONN10.6
D0  (via drill 0.33)
  Top 0.305: 182.88,190.5 194.31,190.5 219.71,165.1 219.71,149.86 U43.4 | 182.88,190.5 182.88,186.69 U35.P15 | 182.88,190.5 179.07,194.31 174.62,194.31 169.54,199.39 119.38,199.39 | 119.38,199.39 U24.A4 | 119.38,199.39 116.84,201.93 v104.14,201.93 | U1.2 8.26,162.56 8.26,150.5 11.43,147.32 13.97,147.32 26.04,135.25 89.53,135.25 U6.3
  Route2 0.305: U7.3 U6.3
  Route15 0.305: v104.14,201.93 96.52,194.31 96.52,142.24 U6.3
D1  (via drill 0.33)
  Top 0.305: U1.1 9.53,163.83 9.53,153.03 11.43,151.13 13.97,151.13 14.61,150.5 14.61,148.59 26.67,136.53 83.19,136.53 U6.6 | U43.5 217.17,149.86 217.17,165.1 194.31,187.96 U35.S16
  Route2 0.305: U7.6 U6.6 | v88.9,193.04 95.25,199.39 114.3,199.39 U24.A3
  Route15 0.305: U6.6 88.9,142.24 v88.9,193.04
  Bottom 0.305: U24.A3 116.84,198.75 117.47,199.39 141.6,199.39 144.15,196.85 161.93,196.85 168.91,189.87 187.32,189.87 U35.S16
D2  (via drill 0.33)
  Top 0.305: U6.10 74.3,137.79 27.3,137.79 15.88,149.22 15.88,160.02 U1.12 | U43.6 214.63,149.86 214.63,165.1 193.04,186.69 187.96,186.69 U35.R16
  Route2 0.305: U6.10 U7.10 | v95.25,196.85 111.76,196.85 U24.B2 115.57,195.58 171.45,195.58 173.99,193.04 184.15,193.04 186.69,190.5 U35.R16
  Route15 0.305: U6.10 78.74,142.24 78.74,172.72 81.28,175.26 81.28,187.96 90.17,196.85 v95.25,196.85
D3  (via drill 0.33)
  Top 0.305: U6.13 67.94,139.06 29.21,139.06 27.94,140.34 27.94,141.6 17.14,152.4 17.14,161.29 U1.13 | U43.7 212.09,149.86 212.09,165.1 193.04,184.15 186.06,184.15 185.42,184.78 185.42,186.69 U35.P16
  Route2 0.305: U6.13 U7.13 | v80.64,189.23 101.6,189.23 102.87,190.5 113.03,190.5 U24.C2 115.57,190.5 137.79,190.5 141.6,194.31 170.18,194.31 172.72,191.77 182.88,191.77 184.15,190.5 U35.P16
  Route15 0.305: U6.13 71.12,142.24 71.12,172.09 79.38,180.34 79.38,187.96 v80.64,189.23
D4  (via drill 0.33)
  Top 0.305: U35.N15 182.88,184.15 182.88,182.25 183.51,181.61 193.04,181.61 209.55,165.1 209.55,149.86 U43.8
  Route2 0.305: U7.16 U6.16 | v77.47,185.42 104.14,185.42 105.41,186.69 U24.E1 113.03,187.96 127,187.96 128.27,189.23 132.08,189.23 133.35,187.96 139.7,187.96 144.78,193.04 168.91,193.04 171.45,190.5 181.61,190.5 182.88,189.23 182.88,186.69 U35.N15
  Route15 0.305: U6.16 63.5,142.24 63.5,179.07 69.85,185.42 v77.47,185.42
  Bottom 0.305: U6.16 57.78,145.41 27.94,145.41 U1.11
D5  (via drill 0.33)
  Top 0.305: U43.9 207.01,149.86 207.01,163.83 191.77,179.07 180.97,179.07 180.34,179.71 180.34,181.61 U35.M14
  Route2 0.305: U7.20 U6.20 | v54.61,177.8 58.42,181.61 109.22,181.61 110.49,182.88 113.03,182.88 U24.F2 116.84,184.15 118.11,185.42 139.7,185.42 146.05,191.77 167.64,191.77 170.18,189.23 179.71,189.23 180.34,188.59 180.34,184.15 U35.M14
  Route15 0.305: v54.61,177.8 54.61,146.05 52.07,143.51 U6.20
  Bottom 0.305: U6.20 48.9,144.15 26.67,144.15 U1.10
D6  (via drill 0.33)
  Top 0.305: U24.H1 113.03,180.34 113.03,182.25 113.67,182.88 120.65,182.88 130.81,193.04 130.81,194.94 131.44,195.58 166.37,195.58 172.72,189.23 180.34,189.23 U35.N16 180.34,186.69 180.34,184.78 179.71,184.15 178.44,184.15 177.8,183.51 177.8,179.07 180.34,176.53 191.77,176.53 204.47,163.83 204.47,149.86 U43.10
  Route2 0.305: U6.23 U7.23 | v45.72,168.91 52.07,175.26 59.69,175.26 63.5,179.07 U24.H1
  Route15 0.305: U6.23 45.72,142.24 v45.72,168.91
  Bottom 0.305: U1.9 25.4,142.88 42.55,142.88 U6.23
D7  (via drill 0.33)
  Top 0.305: U43.11 201.93,149.86 201.93,163.83 191.77,173.99 180.34,173.99 176.53,177.8 175.26,177.8 | 175.26,177.8 170.18,177.8 168.91,179.07 149.86,179.07 148.59,177.8 133.35,177.8 130.81,175.26 113.03,175.26 U24.J1 110.49,175.26 46.99,175.26 v40.64,168.91 | 175.26,177.8 175.26,186.06 175.9,186.69 177.8,186.69 U35.M15
  Route2 0.305: U7.25 U6.25
  Route15 0.305: v40.64,168.91 40.64,146.05 39.37,144.78 U6.25
  Bottom 0.305: U6.25 37.47,139.06 26.04,139.06 12.7,152.4 U1.8
D8  (via drill 0.33)
  Route2 0.305: U8.3 U9.3 | v99.06,167.64 106.05,167.64 109.86,171.45 111.76,171.45 U24.K2 115.57,172.72 141.6,172.72 147.96,179.07 163.19,179.07 165.1,180.97 174.62,180.97 U35.L14
  Route15 0.305: U8.3 99.06,129.54 v99.06,167.64
  Bottom 0.305: U8.3 89.53,131.44 29.21,131.44 27.94,132.72 27.94,135.25 15.88,147.32 10.79,147.32 8.89,145.41 U2.1
D9  (via drill 0.33)
  Route2 0.305: U8.6 U9.6 | v92.71,161.29 93.98,162.56 106.68,162.56 113.03,168.91 116.84,168.91 U24.L4 120.65,170.18 142.88,170.18 144.15,171.45 144.15,172.09 148.59,176.53 172.09,176.53 177.8,182.25 177.8,184.15 U35.L15
  Route15 0.305: U8.6 91.44,129.54 91.44,160.02 v92.71,161.29
  Bottom 0.305: U2.2 8.89,142.88 10.16,144.15 17.14,144.15 24.77,136.53 24.77,133.35 27.94,130.18 83.19,130.18 U8.6
D10  (via drill 0.33)
  Top 0.305: v123.19,201.93 v171.45,201.93
  Route2 0.305: U9.10 U8.10
  Route15 0.305: U8.10 81.28,129.54 v81.28,168.28 | U35.L16 171.45,193.04 v171.45,201.93 | U24.L5 123.19,172.72 v123.19,201.93
  Bottom 0.305: v81.28,168.28 81.28,171.45 82.55,172.72 92.71,172.72 93.98,171.45 93.98,168.91 96.52,166.37 116.84,166.37 U24.L5 | U8.10 74.3,128.91 26.67,128.91 17.78,137.79 16.51,137.79 14.61,139.7 14.61,140.97 U2.13
D11  (via drill 0.33)
  Route2 0.305: U9.13 U8.13 | v73.66,171.45 77.47,175.26 130.81,175.26 U24.H10 135.89,180.34 139.7,180.34 140.97,181.61 147.96,181.61 150.5,184.15 172.72,184.15 U35.K15
  Route15 0.305: U8.13 73.66,129.54 v73.66,171.45
  Bottom 0.305: U2.12 16.51,136.53 17.78,136.53 26.67,127.64 67.94,127.64 U8.13
D12  (via drill 0.33)
  Top 0.305: U2.11 19.68,137.79 28.57,128.91 36.2,128.91 38.1,127 38.1,125.09 39.37,123.83 56.52,123.83 U9.16
  Route2 0.305: U35.K16 172.72,186.69 150.5,186.69 146.69,182.88 135.89,182.88 U24.G10 124.46,181.61 120.65,177.8 105.41,177.8 104.14,176.53 73.66,176.53 v66.04,168.91 | U9.16 U8.16
  Route15 0.305: U8.16 66.04,129.54 v66.04,168.91
D13  (via drill 0.33)
  Top 0.305: U2.10 13.97,136.53 18.41,136.53 27.3,127.64 34.92,127.64 35.56,127 35.56,125.09 38.1,122.56 47.62,122.56 U9.20 | v170.18,200.66 v133.35,200.66
  Route2 0.305: U8.20 U9.20 | v62.23,182.88 80.01,182.88 81.28,184.15 109.22,184.15 110.49,185.42 115.57,185.42 116.84,186.69 U24.E10
  Route15 0.305: U8.20 53.34,127 53.34,142.88 55.88,145.41 55.88,176.53 v62.23,182.88 | v133.35,200.66 133.35,187.96 U24.E10 | U35.J16 170.18,189.23 v170.18,200.66
D14  (via drill 0.33)
  Top 0.305: v168.91,196.85 v138.43,196.85 137.16,198.12 121.28,198.12 120.65,197.49 120.65,196.22 120.02,195.58 84.45,195.58 80.64,191.77 53.34,191.77 48.26,186.69 v48.26,177.16 | U2.9 14.61,130.81 19.05,130.81 28.57,121.28 41.27,121.28 U9.23
  Route2 0.305: U8.23 U9.23
  Route15 0.305: v48.26,177.16 48.26,129.54 U8.23 | v138.43,196.85 138.43,193.04 U24.C11 | U35.H16 v168.91,196.85
D15  (via drill 0.33)
  Top 0.305: U2.8 13.97,128.91 19.05,128.91 27.94,120.02 37.47,120.02 U9.25 | U35.H15 167.64,186.69 167.64,189.23 162.56,194.31 U24.B11
  Route2 0.305: U8.25 U9.25 | v43.18,168.91 43.18,181.61 53.34,191.77 106.68,191.77 107.95,193.04 135.89,193.04 U24.B11
  Route15 0.305: U8.25 43.18,129.54 v43.18,168.91
D16  (via drill 0.33)
  Route2 0.305: U10.3 U11.3 | v124.46,208.28 v153.67,208.28
  Route15 0.305: U10.3 102.87,118.11 v102.87,193.04 | U24.B4 118.11,195.58 118.11,201.93 v124.46,208.28 | U35.G16 166.37,195.58 v153.67,208.28
  Bottom 0.305: U10.3 89.53,116.2 22.86,116.2 17.78,121.28 8.26,121.28 6.99,122.56 U3.1 | v102.87,193.04 118.11,193.04 U24.B4
D17  (via drill 0.33)
  Route2 0.305: U10.6 U11.6
  Route15 0.305: U10.6 93.98,116.84 v93.98,187.96
  Bottom 0.305: U11.6 83.19,107.31 20.95,107.31 20.32,107.95 16.51,107.95 14.61,109.86 14.61,110.49 U3.10 | v93.98,187.96 101.6,195.58 115.57,195.58 U24.B3 118.11,195.58 118.11,197.49 118.75,198.12 140.97,198.12 143.51,195.58 161.29,195.58 165.1,191.77 165.1,186.69 U35.G15
D18  (via drill 0.33)
  Top 0.305: U24.C1 95.25,191.77 v86.36,182.88
  Route2 0.305: U10.10 U11.10
  Route15 0.305: U10.10 80.01,113.03 82.55,113.03 86.36,116.84 v86.36,182.88 | U24.C1 110.49,193.04 110.49,201.93 120.02,211.46 147.96,211.46 163.83,195.58 U35.F16
  Bottom 0.305: U11.10 74.3,106.05 20.32,106.05 19.68,106.68 15.88,106.68 U3.9
D19  (via drill 0.33)
  Route2 0.305: U10.13 U11.13
  Route15 0.305: U10.13 73.66,114.3 81.28,114.3 83.82,116.84 v83.82,182.88
  Bottom 0.305: U11.13 67.94,104.78 19.68,104.78 19.05,105.41 14.61,105.41 U3.8 | v83.82,182.88 86.36,185.42 97.79,185.42 101.6,189.23 U24.D1 113.03,190.5 125.73,190.5 128.27,193.04 128.27,194.94 128.91,195.58 138.43,195.58 139.7,194.31 160.02,194.31 162.56,191.77 162.56,186.69 U35.F15
D20  (via drill 0.33)
  Top 0.305: U10.16 58.42,114.3 25.4,114.3 18.41,121.28 13.97,121.28 U3.13
  Route2 0.305: U10.16 U11.16
  Route15 0.305: U10.16 64.77,107.95 100.33,107.95 104.14,111.76 v104.14,170.18
  Bottom 0.305: U35.E16 161.29,190.5 158.75,193.04 133.35,193.04 132.08,191.77 128.27,191.77 123.19,186.69 U24.E2 113.03,185.42 110.49,185.42 104.14,179.07 v104.14,170.18
D21  (via drill 0.33)
  Top 0.305: U24.G2 121.28,181.61 130.18,190.5 161.29,190.5 162.56,189.23 162.56,184.15 U35.F14
  Route2 0.305: U10.20 U11.20 | v58.42,176.53 62.23,180.34 113.03,180.34 U24.G2
  Route15 0.305: U10.20 58.42,116.84 v58.42,176.53
  Bottom 0.305: U10.20 47.62,114.94 20.32,114.94 19.68,115.57 15.88,115.57 13.97,117.47 U3.12
D22  (via drill 0.33)
  Route2 0.305: U10.23 U11.23
  Route15 0.305: U10.23 48.26,106.68 100.33,106.68 105.41,111.76 v105.41,171.45 | U24.H2 120.65,185.42 120.65,201.93 125.73,207.01 147.32,207.01 160.02,194.31 160.02,186.69 U35.E15
  Bottom 0.305: U24.H2 113.03,177.8 107.95,177.8 105.41,175.26 v105.41,171.45 | U10.23 41.27,113.67 19.68,113.67 19.05,114.3 15.24,114.3 13.34,116.2 10.79,116.2 6.99,120.02 U3.2
D23  (via drill 0.33)
  Route2 0.305: U11.25 U10.25
  Route15 0.305: U10.25 44.45,105.41 100.33,105.41 106.68,111.76 v106.68,170.18
  Bottom 0.305: U35.D16 156.21,190.5 143.51,190.5 140.97,187.96 133.35,187.96 132.08,189.23 128.27,189.23 127,187.96 125.73,187.96 U24.J2 113.03,175.26 107.95,175.26 106.68,173.99 v106.68,170.18 | U10.25 37.47,112.39 19.05,112.39 18.41,113.03 14.61,113.03 U3.11
D24
  Route2 0.305: U12.3 U13.3
  Route15 0.305: U12.3 95.25,96.52 96.52,97.79 100.33,97.79 111.76,109.22 111.76,165.1 114.3,167.64 U24.L2 113.03,172.72 113.03,201.93 120.65,209.55 147.32,209.55 162.56,194.31 162.56,184.15 U35.E14
  Bottom 0.305: U12.3 90.81,99.69 20.95,99.69 20.32,100.33 15.24,100.33 14.61,100.97 6.35,100.97 U4.1
D25  (via drill 0.33)
  Route2 0.305: U12.6 U13.6
  Route15 0.305: U12.6 91.44,99.06 99.69,99.06 107.95,107.31 v107.95,167.64
  Bottom 0.305: U12.6 84.45,98.42 20.32,98.42 19.68,99.06 15.24,99.06 14.61,98.42 6.35,98.42 U4.2 | v107.95,167.64 109.22,168.91 114.3,168.91 U24.L3 118.11,172.72 118.11,176.53 127,185.42 140.97,185.42 144.78,189.23 154.94,189.23 U35.C16
D26
  Route2 0.305: U13.10 U12.10
  Route15 0.305: U24.K4 118.11,172.72 118.11,169.54 113.03,164.47 113.03,102.87 110.49,100.33 109.22,100.33 101.6,92.71 78.74,92.71 77.47,93.98 U12.10
  Bottom 0.305: U12.10 75.56,97.16 19.68,97.16 19.05,97.79 15.88,97.79 15.24,97.16 U4.13 | U24.K4 119.38,175.26 127,182.88 147.32,182.88 148.59,184.15 148.59,186.06 150.5,187.96 U35.B16
D27
  Top 0.305: U24.G11 147.32,181.61 149.86,184.15 154.94,184.15 U35.C15 | U12.13 67.31,92.71 14.61,92.71 U4.12
  Route2 0.305: U13.13 U12.13
  Route15 0.305: U12.13 73.66,91.44 101.6,91.44 109.22,99.06 110.49,99.06 114.3,102.87 114.3,163.83 116.2,165.74 126.36,165.74 130.81,170.18 130.81,175.26 133.35,177.8 133.35,179.71 133.99,180.34 135.89,180.34 U24.G11
D28
  Top 0.305: U24.F10 135.89,185.42 148.59,185.42 149.86,186.69 152.4,186.69 U35.B15 | U13.16 58.42,91.44 13.34,91.44 U4.11
  Route2 0.305: U13.16 U12.16
  Route15 0.305: U24.F10 135.89,182.88 138.43,182.88 139.7,181.61 139.7,171.45 133.35,165.1 133.35,161.29 128.27,156.21 128.27,154.31 125.73,151.76 125.73,149.22 120.65,144.15 119.38,144.15 118.11,142.88 118.11,140.34 115.57,137.79 115.57,102.87 110.49,97.79 109.22,97.79 101.6,90.17 67.31,90.17 U12.16
D29
  Top 0.305: U13.20 48.26,83.82 13.34,83.82 U4.8 | U24.E11 140.97,186.69 142.24,187.96 151.13,187.96 152.4,189.23 156.84,189.23 157.48,188.59 157.48,184.15 U35.C14
  Route2 0.305: U12.20 U13.20
  Route15 0.305: U13.20 54.61,85.09 101.6,85.09 109.22,92.71 110.49,92.71 116.84,99.06 116.84,136.53 120.02,139.7 134.62,139.7 136.53,141.6 136.53,164.47 140.97,168.91 140.97,182.88 U24.E11
D30
  Top 0.305: U24.D10 133.35,187.96 133.35,180.97 133.99,180.34 148.59,180.34 149.86,181.61 152.4,181.61 U35.B14 | U13.23 41.91,85.09 14.61,85.09 U4.9
  Route2 0.305: U13.23 U12.23
  Route15 0.305: U24.D10 135.89,187.96 142.24,187.96 143.51,186.69 143.51,168.28 140.97,165.74 140.97,142.24 137.16,138.43 120.65,138.43 118.11,135.89 118.11,99.06 110.49,91.44 109.22,91.44 101.6,83.82 48.26,83.82 U13.23
D31
  Top 0.305: U13.25 36.83,90.17 13.34,90.17 U4.10
  Route2 0.305: U12.25 U13.25
  Route15 0.305: U24.C10 135.89,190.5 142.24,190.5 144.78,187.96 144.78,154.94 142.24,152.4 142.24,142.24 137.16,137.16 120.65,137.16 119.38,135.89 119.38,99.06 110.49,90.17 109.22,90.17 101.6,82.55 44.45,82.55 U13.25
  Bottom 0.305: U24.C10 135.89,190.5 140.97,190.5 142.24,191.77 157.48,191.77 160.02,189.23 160.02,179.07 U35.D12
DCD0
  Top 0.305: U47.6 196.85,59.69 215.9,59.69 CONN3.1
DCD1
  Top 0.305: U49.6 196.85,24.13 215.9,24.13 CONN4.1
DCD2
  Top 0.305: U51.6 231.14,59.69 250.19,59.69 CONN5.1
DCD3
  Top 0.305: U53.6 231.14,24.13 250.19,24.13 CONN6.1
DCD4
  Bottom 0.305: U54.6 265.43,57.15 284.48,57.15 CONN7.1
DCD5
  Top 0.305: U56.6 265.43,24.13 284.48,24.13 CONN8.1
DCD6
  Top 0.305: U59.6 299.72,59.69 318.77,59.69 CONN9.1
DCD7
  Top 0.305: U61.6 299.72,24.13 318.77,24.13 CONN10.1
DRQ
  Route15 0.305: U38.7 157.48,109.22 157.48,101.6 158.75,100.33 225.43,100.33 230.5,95.25 237.49,95.25 U50.5
DRQS  (via drill 0.33)
  Top 0.305: U40.18 177.8,54.61 177.8,64.77 184.15,71.12 v184.15,93.98
  Route15 0.305: U50.4 238.76,93.98 v184.15,93.98
DRQS0
  Route15 0.305: U41.23 167.64,44.45 167.64,52.07 U40.3
DRQS1  (via drill 0.33)
  Route2 0.305: U57.25 276.86,80.01 276.86,74.93 274.32,72.39 v274.32,63.5
  Bottom 0.305: U40.4 175.26,62.23 186.69,62.23 187.96,63.5 v274.32,63.5
DTR0
  Top 0.305: U47.5 203.2,53.34 212.09,53.34 214.63,50.8 CONN3.7
DTR1
  Top 0.305: U49.5 203.2,17.78 CONN4.7
DTR2
  Top 0.305: U51.5 237.49,53.34 246.38,53.34 248.92,50.8 CONN5.7
DTR3
  Top 0.305: U53.5 237.49,17.78 CONN6.7
DTR4
  Top 0.305: U54.5 271.78,53.34 280.67,53.34 283.21,50.8 CONN7.7
DTR5
  Top 0.305: U56.5 271.78,17.78 CONN8.7
DTR6
  Top 0.305: U59.5 306.07,53.34 314.96,53.34 317.5,50.8 CONN9.7
DTR7
  Top 0.305: U61.5 306.07,17.78 CONN10.7
DUACLK  (via drill 0.33)
  Route2 0.305: U58.8 304.8,97.16 R6.1 307.34,57.78 304.17,54.61 v299.72,54.61 | U52.36 233.68,44.45 233.68,46.35 233.04,46.99 229.24,46.99 226.06,50.16 226.06,59.05 229.24,62.23 232.41,62.23 234.31,64.14 234.31,65.41 233.04,66.67 230.5,66.67 U46.32
  Route15 0.305: v299.72,54.61 297.18,54.61 294.64,52.07 294.64,45.72 293.37,44.45 270.51,44.45 U55.36 267.97,44.45 236.22,44.45 U52.36 233.68,44.45 201.93,44.45 U48.36
DUART_X1
  Route2 0.305: C75.1 326.39,42.55 326.39,41.91 | 326.39,41.91 X1.1 | 326.39,41.91 304.8,41.91 U60.36
  Bottom 0.305: C75.1 324.49,49.53 324.49,64.14 311.15,77.47 311.15,97.79 U58.9
DUART_X2
  Route2 0.305: U60.37 302.26,44.45 302.26,41.91 307.34,36.83 323.21,36.83 X1.2
  Bottom 0.305: C77.1 326.39,29.84 X1.2
FB1
  Route15 0.305: U50.10 235.59,90.81 239.4,90.81 U50.13
GND  (via drill 3.6)
  Bottom 0.305: U30.7 123.83,99.69 128.91,99.69 U29.13 U29.14
  other vias: 20.32,76.23 332.74,76.23
  pour Top (rank 6, no thermals): 14.61,81.92 26.04,81.92 26.04,70.48 14.61,70.48
  pour Top (rank 6, no thermals): 327.02,81.92 338.45,81.92 338.45,70.48 327.02,70.48
  pour Ground (rank 6): 0,215.9 0,58.42 12.7,58.42 12.7,0 342.9,0 342.9,215.9
  pour Bottom: 14.61,81.92 14.61,70.48 26.04,70.48 26.04,81.92
  pour Bottom: 327.02,81.92 327.02,70.48 338.45,70.48 338.45,81.92
HSAC
  Bottom 0.305: U30.6 125.09,98.42 146.05,98.42 149.86,94.61 168.91,94.61 170.18,95.89 170.18,97.79 172.72,100.33 172.72,137.16 U36.1
IO0
  Bottom 0.305: CONN15.A10 294.64,149.86 293.37,151.13 293.37,163.83 294.64,165.1 CONN14.A10 294.64,170.18 293.37,171.45 293.37,184.15 294.64,185.42 CONN13.A10 294.64,190.5 293.37,191.77 293.37,204.47 294.64,205.74 CONN12.A10
IO1
  Bottom 0.305: CONN15.A9 297.18,149.86 295.91,151.13 295.91,163.83 297.18,165.1 CONN14.A9 297.18,170.18 295.91,171.45 295.91,184.15 297.18,185.42 CONN13.A9 297.18,190.5 295.91,191.77 295.91,204.47 297.18,205.74 CONN12.A9
IO2
  Bottom 0.305: CONN15.A8 299.72,149.86 298.45,151.13 298.45,163.83 299.72,165.1 CONN14.A8 299.72,170.18 298.45,171.45 298.45,184.15 299.72,185.42 CONN13.A8 299.72,190.5 298.45,191.77 298.45,204.47 299.72,205.74 CONN12.A8
IO3
  Bottom 0.305: CONN15.A7 302.26,149.86 300.99,151.13 300.99,163.83 302.26,165.1 CONN14.A7 302.26,170.18 300.99,171.45 300.99,184.15 302.26,185.42 CONN13.A7 302.26,190.5 300.99,191.77 300.99,204.47 302.26,205.74 CONN12.A7
IO4
  Route2 0.305: CONN12.A6 304.8,205.74 303.53,204.47 303.53,191.77 304.8,190.5 CONN13.A6 304.8,185.42 303.53,184.15 303.53,171.45 304.8,170.18 CONN14.A6 304.8,165.1 303.53,163.83 303.53,151.13 304.8,149.86 CONN15.A6
IO5
  Route2 0.305: CONN12.A5 307.34,205.74 306.07,204.47 306.07,191.77 307.34,190.5 CONN13.A5 307.34,185.42 306.07,184.15 306.07,171.45 307.34,170.18 CONN14.A5 307.34,165.1 306.07,163.83 306.07,151.13 307.34,149.86 CONN15.A5
IO6
  Route2 0.305: CONN12.A4 309.88,205.74 308.61,204.47 308.61,191.77 309.88,190.5 CONN13.A4 309.88,185.42 308.61,184.15 308.61,171.45 309.88,170.18 CONN14.A4 309.88,165.1 308.61,163.83 308.61,151.13 309.88,149.86 CONN15.A4
IO7
  Route2 0.305: CONN12.A3 312.42,205.74 311.15,204.47 311.15,191.77 312.42,190.5 CONN13.A3 312.42,185.42 311.15,184.15 311.15,171.45 312.42,170.18 CONN14.A3 312.42,165.1 311.15,163.83 311.15,151.13 312.42,149.86 CONN15.A3
IO8
  Route15 0.305: CONN12.A2 314.96,205.74 313.69,204.47 313.69,191.77 314.96,190.5 CONN13.A2 314.96,185.42 313.69,184.15 313.69,171.45 314.96,170.18 CONN14.A2 314.96,165.1 313.69,163.83 313.69,151.13 314.96,149.86 CONN15.A2
IO9
  Route2 0.305: CONN12.A1 317.5,205.74 316.23,204.47 316.23,191.77 317.5,190.5 CONN13.A1 317.5,185.42 316.23,184.15 316.23,171.45 317.5,170.18 CONN14.A1 317.5,165.1 316.23,163.83 316.23,151.13 317.5,149.86 CONN15.A1
N$1
  cutout Power: 31.75,208.28 31.75,203.2 62.23,203.2 62.23,208.28
N$25
  cutout Ground: 31.75,208.28 62.23,208.28 62.23,203.2 31.75,203.2
PA0
  Bottom 0.305: RES15.8 165.1,17.78 165.1,21.59 U41.49
PA1
  Bottom 0.305: RES16.8 167.64,15.24 167.64,19.05 U41.50
PA2
  Bottom 0.305: RES15.6 171.45,17.14 170.18,18.41 170.18,21.59 U41.51
PA3
  Top 0.305: U41.52 170.18,19.05 170.18,15.24 RES16.6
PA4
  Bottom 0.305: RES15.4 176.53,17.14 175.26,18.41 173.35,18.41 172.72,19.05 172.72,21.59 U41.53
PA5
  Top 0.305: U41.54 175.26,19.05 175.26,15.24 RES16.4
PA6
  Bottom 0.305: RES15.2 179.07,19.05 175.9,19.05 175.26,19.68 175.26,21.59 U41.55
PA7
  Top 0.305: RES16.2 180.34,15.24 180.34,17.78 179.71,18.41 178.44,18.41 U41.56
PDI0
